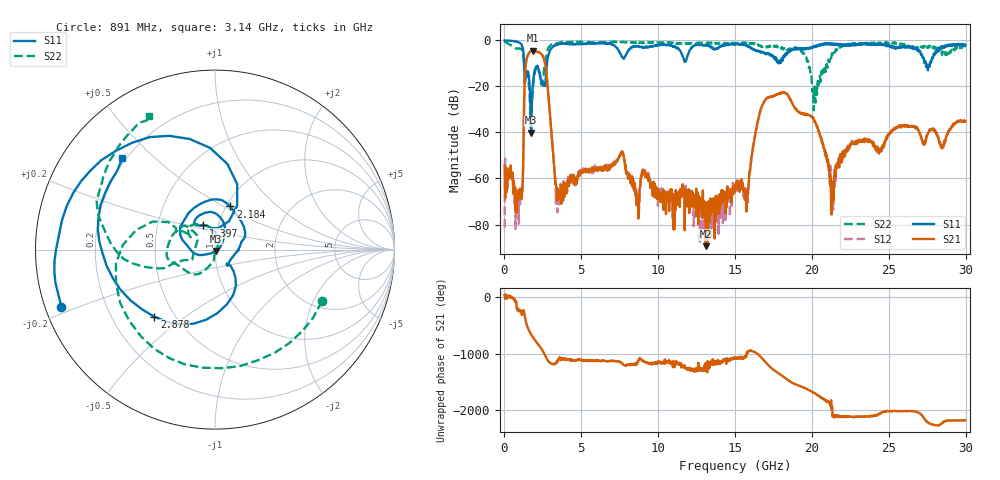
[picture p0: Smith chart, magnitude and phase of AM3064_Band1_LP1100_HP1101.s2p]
# Hz S DB R 50.0
!freq dBS11 angS11 dBS21 angS21 dBS12 angS12 dBS22 angS22
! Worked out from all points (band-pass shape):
!   1600 points, 10 MHz to 29.98 GHz, reference 50 ohm
!   highest |S21| = -4.48 dB at 1.828 GHz (marker M1); lowest = -89.4 dB at 13.09 GHz (marker M2)
!   |S21| within 3 dB of the highest: 1.468 GHz to 2.537 GHz (1.07 GHz wide, 53.4 % of centre)
!   lowest |S11| = -40.2 dB at 1.734 GHz (marker M3), VSWR 1.02, Z = 50.5 - j0.831 ohm
!   |S11| at or under -10 dB: 1.277 GHz to 2.767 GHz (1.49 GHz wide, 73.7 % of centre); 17.84769 GHz to 17.8564 GHz (8.706 MHz wide, 0.0488 % of centre); 27.4 GHz to 27.68 GHz (281.6 MHz wide, 1.02 % of centre)
!   |S22| runs from -40.9 to -0.5 dB; largest |S21 - S12| = 0.0087
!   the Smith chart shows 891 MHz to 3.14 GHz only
!   S11 on the Smith chart (normalised r, x): 891 MHz: 0.05, -0.18; 1.397 GHz: 0.84, +0.23; 2.184 GHz: 1.05, +0.54; 2.878 GHz: 0.39, -0.39; 3.14 GHz: 0.19, +0.40
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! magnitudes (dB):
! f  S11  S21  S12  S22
! 10 MHz  -0.1  -54.4  -81.3  -0.5
! 891 MHz  -0.8  -65.5  -65.0  -3.6
! 1.116 GHz  -1.9  -68.2  -68.5  -3.9
! 1.397 GHz  -16.4  -10.0  -9.9  -16.1
! 1.734 GHz  -40.2  -4.7  -4.6  -40.9
! 1.828 GHz  -20.7  -4.5  -4.5  -22.3
! 2.184 GHz  -11.9  -5.1  -5.1  -12.2
! 2.878 GHz  -6.0  -25.6  -25.6  -3.0
! 3.14 GHz  -2.8  -46.8  -46.8  -1.6
! 3.478 GHz  -1.8  -68.7  -68.3  -1.2
! 5.015 GHz  -1.4  -56.7  -56.1  -0.6
! 7.62 GHz  -6.9  -49.1  -48.9  -0.7
! 8.613 GHz  -2.6  -69.7  -68.4  -0.9
! 10 GHz  -2.1  -69.1  -65.6  -0.9
! 13.09 GHz  -2.0  -89.4  -70.9  -1.0
! 15 GHz  -1.7  -62.8  -65.7  -1.3
! 15.72 GHz  -2.3  -67.6  -72.5  -1.3
! 17.05 GHz  -5.6  -25.3  -25.2  -3.1
! 19.99 GHz  -3.4  -33.2  -33.1  -17.8
! 21.3 GHz  -1.8  -70.5  -69.2  -5.7
! 25 GHz  -2.0  -41.0  -40.8  -1.2
! 29.98 GHz  -1.9  -35.1  -35.3  -3.0
